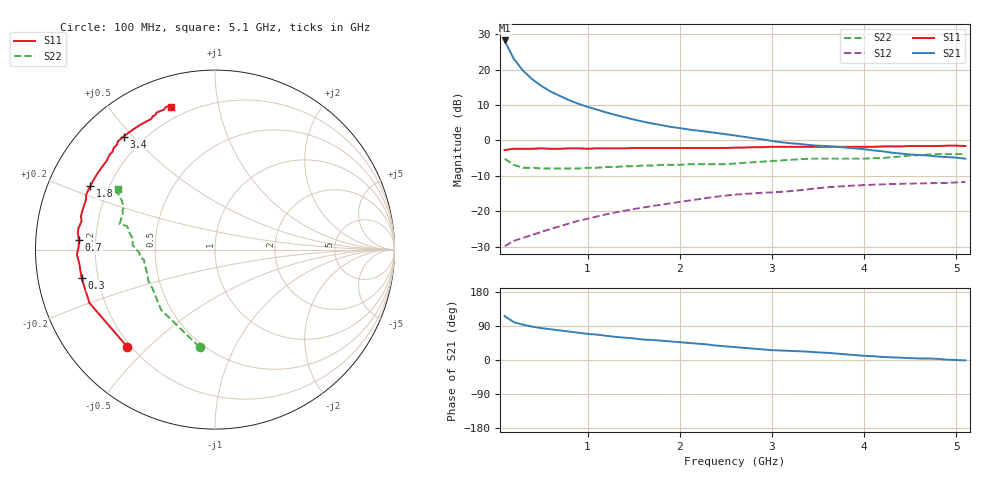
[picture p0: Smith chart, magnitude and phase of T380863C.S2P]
!AT-38086
!S-PARAMETERS at Vce=3.6V  Ic=80mA.  LAST UPDATED 08-05-96
# ghz s ma r 50
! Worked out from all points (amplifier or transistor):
!   51 points, 100 MHz to 5.1 GHz, reference 50 ohm
!   highest |S21| = 28.2 dB at 100 MHz (marker M1)
!   |S21| within 3 dB of that: start of sweep to 157.7 MHz
!   unconditionally stable (mu >= 1): 855 MHz to end of sweep
!   at 900 MHz: K = 1.01, MAG = 15.8 dB, |S12| = -22.7 dB
!   at 2.6 GHz: K = 1.10, MAG = 6.4 dB, |S12| = -15.3 dB
!   at 5.1 GHz: K = 1.11, MAG = 1.3 dB, |S12| = -11.8 dB
!   S11 on the Smith chart (normalised r, x): 100 MHz: 0.19, -0.43; 300 MHz: 0.14, -0.10; 700 MHz: 0.14, +0.03; 1.8 GHz: 0.13, +0.24; 3.4 GHz: 0.13, +0.47; 5.1 GHz: 0.14, +0.73
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0.1  0.73 -132.0  25.72 116.0  0.032 38.0  0.55 -99.0
0.2  0.76 -157.0  14.14 100.0  0.038 34.0  0.45 -132.0
0.3  0.76 -168.0  9.61 93.0  0.042 38.0  0.41 -148.0
0.4  0.76 -174.0  7.28 88.0  0.046 41.0  0.41 -155.0
0.5  0.77 -178.0  5.86 84.0  0.051 45.0  0.4 -160.0
0.6  0.76 179.0  4.88 81.0  0.056 48.0  0.4 -164.0
0.7  0.76 176.0  4.23 78.0  0.061 50.0  0.4 -167.0
0.8  0.77 173.0  3.7 75.0  0.067 52.0  0.4 -169.0
0.9  0.77 171.0  3.28 72.0  0.073 53.0  0.4 -172.0
1  0.76 168.0  2.97 69.0  0.078 54.0  0.41 -173.0
1.2  0.77 163.0  2.48 64.0  0.09 56.0  0.42 -176.0
1.3  0.77 161.0  2.29 61.0  0.096 56.0  0.42 -177.0
1.6  0.78 155.0  1.84 54.0  0.112 56.0  0.44 180.0
1.8  0.78 153.0  1.64 51.0  0.123 56.0  0.45 178.0
2.1  0.78 149.0  1.42 45.0  0.141 56.0  0.46 177.0
2.6  0.79 138.0  1.17 34.0  0.171 52.0  0.47 171.0
3  0.81 132.0  0.98 26.0  0.184 49.0  0.51 165.0
3.4  0.81 129.0  0.86 22.0  0.204 48.0  0.55 165.0
3.5  0.81 128.0  0.84 20.0  0.211 48.0  0.55 165.0
3.8  0.81 122.0  0.79 15.0  0.226 44.0  0.55 163.0
4.3  0.82 114.0  0.67 7.0  0.241 38.0  0.58 153.0
5.1  0.83 107.0  0.55 -1.0  0.258 33.0  0.64 148.0
